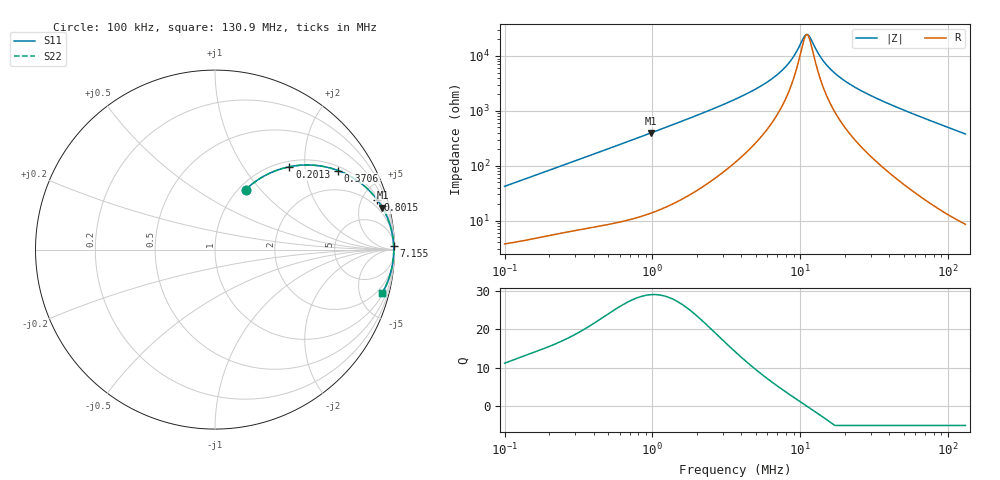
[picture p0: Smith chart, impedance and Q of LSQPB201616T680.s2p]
! LSQPB201616T680  S-PARAMETER MODEL  ( General Type )
! Model Generated by TAIYO YUDEN Corporation (http://www.ty-top.com)
! Version 2.0
! TAIYO YUDEN Control No. 100810NC14SB-FKC
! Copyright(c) 2008 TAIYO YUDEN CO.,LTD. All Rights Reserved.
! Product Description (link to TY-COMPAS)
! https://ds.yuden.co.jp/TYCOMPAS/or/detail?pn=LSQPB201616T680K&u=M
! Products Name : Inductors
! Characteristics :
!  Inductance : 68 uH , SRF(min) : 8.0 MHz , DC Resistance(max) : 3.64 Ohm
!  Rated Current : Saturation :200 mA , Temp Rise : 190 mA (40 degC)
!  Case Size : 2.0 x 1.6 / 0.079 x 0.063 [mm/inch] , Thickness : 1.6 / 0.063 [mm/inch]
!  (Conditions: Temperature = 25 degC , DC Bias Current/Voltage = 0A / 0V)
! External Node Assignments :
!  1  o---GGG---o  2
! GND o---------o GND
! Frequency Range : 0.1MHz  -  130.914307MHz  [ 402 STEP ]
# MHz S RI R 50
! Freq[MHz].  S11 Real  S11 Imag  S21 Real  S21 Imag  S12 Real  S12 Imag  S22 Real  S22 Imag
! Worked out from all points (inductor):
!   401 points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, 100 kHz to 130.9 MHz, reference 50 ohm
!   read as one part in series: L = 66.4 uH near 103.7 kHz
!   highest Q = 29 at 976.4 kHz (marker M1), where L = 64.4 uH
!   self-resonance near 11.01 MHz
!   S11 on the Smith chart (normalised r, x): 100 kHz: 1.08, +0.84; 201.3 kHz: 1.11, +1.66; 370.6 kHz: 1.15, +3.01; 801.5 kHz: 1.23, +6.48; 7.155 MHz: 20, +95; 130.9 MHz: 1.17, -7.58
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0.1  0.1714 0.3347  0.8286 -0.3347  0.8286 -0.3347  0.1714 0.3347
0.138122  0.2652 0.4051  0.7348 -0.4051  0.7348 -0.4051  0.2652 0.4051
0.201329  0.4147 0.4615  0.5853 -0.4615  0.5853 -0.4615  0.4147 0.4615
0.332733  0.6414 0.4547  0.3586 -0.4547  0.3586 -0.4547  0.6414 0.4547
0.370553  0.6865 0.4404  0.3135 -0.4404  0.3135 -0.4404  0.6865 0.4404
0.540122  0.8174 0.3666  0.1826 -0.3666  0.1826 -0.3666  0.8174 0.3666
0.801542  0.9051 0.276  0.0949 -0.276  0.0949 -0.276  0.9051 0.276
0.976435  0.9328 0.2337  0.0672 -0.2337  0.0672 -0.2337  0.9328 0.2337
1.10711  0.9462 0.2089  0.0538 -0.2089  0.0538 -0.2089  0.9462 0.2089
3.683715  0.9921 0.0595  0.00788 -0.0595  0.00788 -0.0595  0.9921 0.0595
5.466638  0.9947 0.0342  0.00531 -0.0342  0.00531 -0.0342  0.9947 0.0342
7.154962  0.9955 0.0202  0.00448 -0.0202  0.00448 -0.0202  0.9955 0.0202
8.716146  0.9958 0.0108  0.00416 -0.0108  0.00416 -0.0108  0.9958 0.0108
10.81021  0.996 0.00113  0.00403 -0.00113  0.00403 -0.00113  0.996 0.00113
11.40805  0.996 -0.00128  0.00402 0.00128  0.00402 0.00128  0.996 -0.00128
12.03896  0.996 -0.00368  0.00403 0.00368  0.00403 0.00368  0.996 -0.00368
13.16895  0.9959 -0.00772  0.00408 0.00772  0.00408 0.00772  0.9959 -0.00772
14.40501  0.9958 -0.0118  0.00416 0.0118  0.00416 0.0118  0.9958 -0.0118
17.86583  0.9955 -0.0221  0.00451 0.0221  0.00451 0.0221  0.9955 -0.0221
24.67673  0.9944 -0.0396  0.00562 0.0396  0.00562 0.0396  0.9944 -0.0396
40.05754  0.9903 -0.074  0.00969 0.074  0.00969 0.074  0.9903 -0.074
130.9143  0.9302 -0.2438  0.0698 0.2438  0.0698 0.2438  0.9302 -0.2438
